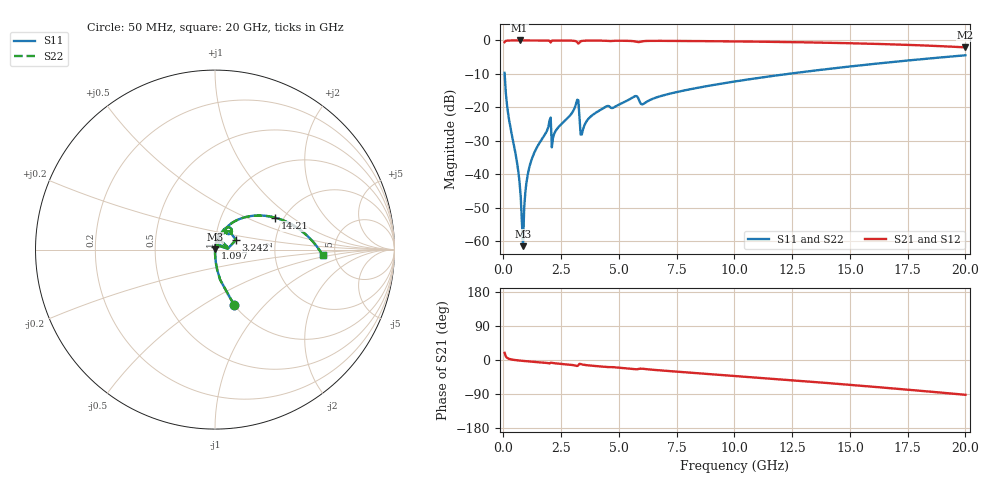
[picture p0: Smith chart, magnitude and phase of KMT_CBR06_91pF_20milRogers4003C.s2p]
! Data measured by Modelithics Inc. support@modelithics.com 813-866-6335
! KEMET CBR0603 91pF, Pad Width= 0.851mm, Pad Length= 0.64mm, Pad Gap= 0.62mm, 20mil Rogers 4003C substrate Data, January 2022
# hz S ma R 50
! 2 Port Network Data from SP1.SP block
! freq  magS11  angS11  magS21  angS21  magS12  angS12  magS22  angS22
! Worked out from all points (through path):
!   401 points, 50 MHz to 20 GHz, reference 50 ohm
!   highest |S21| = 0.00 dB at 698.4 MHz (marker M1); lowest = -2.1 dB at 20 GHz (marker M2)
!   group delay of S21, straight-line fit = 12.8 ps
!   lowest |S11| = -61.4 dB at 848 MHz (marker M3), VSWR 1.00, Z = 50.1 + j0.0656 ohm
!   |S11| at or under -10 dB: 52.8 MHz to 12.31 GHz (12.26 GHz wide, 198 % of centre)
!   |S22| runs from -61.4 to -4.4 dB; largest |S21 - S12| = 0
!   S11 on the Smith chart (normalised r, x): 50 MHz: 1.00, -0.69; 1.097 GHz: 1.00, +0.02; 3.242 GHz: 1.26, +0.14; 14.21 GHz: 1.81, +0.75; 20 GHz: 3.97, -0.37
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5e7  0.3282 -70.9  0.9443 19.0  0.9443 19.0  0.3282 -70.9
2.495e8  0.06355 -86.8  0.9977 2.9  0.9977 2.9  0.06355 -86.8
5.4875e8  0.01811 -89.2  0.9994 -0.5  0.9994 -0.5  0.01811 -89.2
6.98375e8  0.007546 -88.0  0.9995 -1.5  0.9995 -1.5  0.007546 -88.0
7.4825e8  0.004629 -85.9  0.9995 -1.8  0.9995 -1.8  0.004629 -85.9
8.48e8  0.0008472 50.7  0.9995 -2.4  0.9995 -2.4  0.0008472 50.7
8.97875e8  0.003143 77.7  0.9994 -2.7  0.9994 -2.7  0.003143 77.7
9.97625e8  0.007638 82.6  0.9994 -3.2  0.9994 -3.2  0.007638 82.6
1.097375e9  0.01183 83.4  0.9993 -3.8  0.9993 -3.8  0.01183 83.4
1.34675e9  0.0215 83.2  0.9991 -5.0  0.9991 -5.0  0.0215 83.2
1.94525e9  0.05131 78.6  0.996 -8.4  0.996 -8.4  0.05131 78.6
2.194625e9  0.04024 79.1  0.9974 -8.5  0.9974 -8.5  0.04024 79.1
3.14225e9  0.1128 63.5  0.9716 -15.2  0.9716 -15.2  0.1128 63.5
3.242e9  0.1285 24.8  0.8962 -13.7  0.8962 -13.7  0.1285 24.8
3.391625e9  0.03948 52.8  0.9822 -11.6  0.9822 -11.6  0.03948 52.8
4.439e9  0.1027 67.8  0.9877 -18.3  0.9877 -18.3  0.1027 67.8
6.73325e9  0.1449 61.5  0.9857 -27.1  0.9857 -27.1  0.1449 61.5
1.0025e10  0.2443 47.4  0.9671 -42.0  0.9671 -42.0  0.2443 47.4
1.336662e10  0.3513 31.9  0.9328 -57.6  0.9328 -57.6  0.3513 31.9
1.42145e10  0.3805 27.8  0.921 -61.7  0.921 -61.7  0.3805 27.8
1.670825e10  0.4713 15.2  0.8765 -74.2  0.8765 -74.2  0.4713 15.2
2e10  0.6002 -2.9  0.7885 -91.9  0.7885 -91.9  0.6002 -2.9
